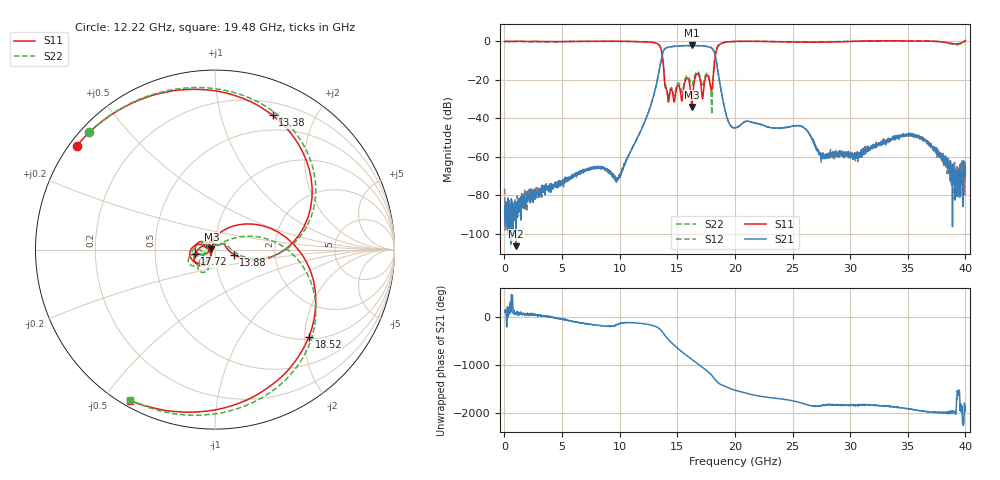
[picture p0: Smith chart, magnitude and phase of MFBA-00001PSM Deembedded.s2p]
!Keysight Technologies,N5247B,US58420632,A.15.75.19
!Date: Thursday, September 22, 2022 11:07:44
!Correction: S11(C  2-Port  )
!S41(C  2-Port  )
!S14(C  2-Port  )
!S44(C  2-Port  )
!S2P File: Measurements: S11, S41, S14, S44:
# Hz S  dB  R 50
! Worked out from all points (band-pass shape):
!   2000 points, 20 MHz to 40 GHz, reference 50 ohm
!   highest |S21| = -2.23 dB at 16.24 GHz (marker M1); lowest = -106.3 dB at 1.02 GHz (marker M2)
!   |S21| within 3 dB of the highest: 13.79 GHz to 18.18 GHz (4.391 GHz wide, 27.5 % of centre)
!   lowest |S11| = -34.2 dB at 16.26 GHz (marker M3), VSWR 1.04, Z = 48.1 + j0.13 ohm
!   |S11| at or under -10 dB: 13.76 GHz to 18.25 GHz (4.496 GHz wide, 28.1 % of centre)
!   |S22| runs from -38.0 to 0.1 dB; largest |S21 - S12| = 0.0011
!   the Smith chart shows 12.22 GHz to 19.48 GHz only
!   S11 on the Smith chart (normalised r, x): 12.22 GHz: 0.02, +0.33; 13.38 GHz: 0.33, +1.47; 13.88 GHz: 1.23, -0.07; 17.72 GHz: 0.80, -0.04; 18.52 GHz: 1.06, -2.10; 19.48 GHz: 0.02, -0.59
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2e7  -0.16 -0.4  -89.23 134.1  -76.55 -106.8  -0.11 -0.4
1.02e9  -0.08 -13.3  -106.33 81.8  -92.41 6.8  -0.14 -13.7
6.7e9  -0.12 -97.5  -67.71 -118.4  -67.80 -123.3  -0.09 -101.2
9.88e9  -0.03 -165.7  -71.53 -145.4  -71.16 -144.4  -0.14 -168.3
1.222e10  -0.32 143.0  -41.26 -140.6  -41.24 -140.9  -0.37 136.9
1.336e10  -1.68 69.5  -17.53 136.6  -17.53 136.6  -1.62 65.5
1.338e10  -1.79 66.8  -16.91 133.4  -16.91 133.4  -1.72 63.0
1.388e10  -19.29 -14.6  -4.25 -3.9  -4.25 -4.0  -17.96 -10.9
1.456e10  -25.77 103.1  -2.80 174.4  -2.80 174.4  -24.79 103.1
1.498e10  -23.67 160.4  -2.56 81.9  -2.56 81.9  -22.33 159.6
1.546e10  -29.28 -166.7  -2.36 -13.6  -2.35 -13.6  -25.71 -172.0
1.624e10  -32.70 158.1  -2.23 -155.9  -2.23 -155.9  -22.77 -166.8
1.626e10  -34.17 176.0  -2.23 -159.5  -2.23 -159.5  -22.84 -162.4
1.692e10  -18.39 171.8  -2.36 84.0  -2.36 84.0  -17.15 -166.8
1.772e10  -18.80 -168.1  -2.91 -70.0  -2.91 -70.0  -17.83 -137.5
1.852e10  -2.93 -42.7  -15.27 74.0  -15.26 74.0  -2.39 -47.6
1.948e10  -0.32 -119.3  -42.25 -37.7  -42.21 -37.9  -0.34 -119.4
2.002e10  -0.09 -134.3  -44.96 -88.0  -44.88 -87.4  -0.22 -138.6
2.35e10  -0.27 160.4  -45.10 107.9  -45.10 107.6  -0.19 156.7
2.668e10  -0.53 90.1  -50.55 -52.8  -50.36 -53.4  -0.45 76.9
3.334e10  0.20 26.3  -51.41 -56.7  -52.65 -68.1  0.05 15.3
4e10  0.37 11.2  -65.38 -74.0  -69.69 73.1  0.08 3.1
